FUNCTION_BLOCK "FB_Betr_Std_Zaehl"
TITLE =Betriebsstundenzähler
//KNOW_HOW_PROTECT
//KNOW_HOW_PROTECT
//
//Autor: Ronald Kleißler
//Stand: August 2005
//
//*******************************************************************************
//Eingänge:
//
//Reset:               Setzt den "Btr_Std_Zaehl" auf Null
//Start_Stop:          Startet bzw. stopt den "Btr_Std_Zaehl"
//Takt_MB_aus_der_CPU: Hier wird das MB aus der HW Konfig. der CPU eintragen
//
//Ausgang:
//
//Betr_STD_Zaehler:    Es wird ein DWORD Speicherbereich benötigt
//*******************************************************************************
AUTHOR : 'Kleißler'
NAME : Bter_Std
VERSION : 0.1


VAR_INPUT
  Reset : BOOL ;
  Start_Stop : BOOL ;
  Takt_MB_aus_der_CPU : BYTE ;
END_VAR
VAR_OUTPUT
  Betr_STD_Zaehler : DWORD ;
END_VAR
VAR
  Flankenmerker : BYTE ;
  Minutenimpuls : BOOL ;
  Stundenimpuls : BOOL ;
  Sekunden : INT ;
  Minuten : INT ;
END_VAR
VAR_TEMP
  TEMP0 : BYTE ;
END_VAR
BEGIN
NETWORK
TITLE =Betriebsstundenzähler rücksetzen

      U     #Start_Stop; //*** Betr. Std. Zaehler reseten ***
      SPBN  M100;
      L     0;
      T     #Betr_STD_Zaehler;
      T     #Minuten;
      T     #Sekunden;
      BEB   ;
M100: NOP   0;
NETWORK
TITLE =Betriebsstundenzähler starten bzw. stoppen

      U     #Reset; //*** Betr. Std. Zaehler starten ***
      SPBN  M601;
NETWORK
TITLE =Impuls bilden aus HW Takt
//Erkennung der positiven Flanken des HW Taktes durch die
//XOW (EXKLUSIV-ODER-Wort 16Bit)
//und die UW (UND-Wort 16 Bit) Verknüpfung
      L     #Takt_MB_aus_der_CPU; //Flankenbildung des HW Taktes
      L     #Flankenmerker;
      XOW   ; //XOW Erkennt den Signalwechsel
      UW    ; //UW bildet die Flanke des MB
      T     #TEMP0;
      TAK   ; //Ergebniss aus AKKU 2 nach AKKU 1
      T     #Flankenmerker;
NETWORK
TITLE =Minuten -  Takt
//Addition des Sekundentakt bis 60
      UN    L      0.4; //Flankenpuls einer Sekunden
      SPB   M400; //wenn nein dann Sprung
      L     #Sekunden; //wenn ja dann addition
      +     1;
      T     #Sekunden;
M400: L     #Sekunden; //60 Sekunden erreicht ?
      L     60;
      >=I   ;
      =     #Minutenimpuls; //wenn ja dann plus 1 Minute
      SPBN  M401; //wenn nein dann Spung
      L     0; //wenn ja dann loesche Sekundenzaehler
      T     #Sekunden;
M401: NOP   0;
NETWORK
TITLE =Stunden -  Takt
//Addition des Minutentakt bis 60
      UN    #Minutenimpuls; //Flankenpuls einer Minute
      SPB   M500; //wenn nein dann Sprung
      L     #Minuten; //wenn ja dann addition
      +     1;
      T     #Minuten;
M500: L     #Minuten; //60 Minuten erreicht ?
      L     60;
      >=I   ;
      =     #Stundenimpuls; //wenn ja dann plus 1 Stunde
      SPBN  M501; //wenn nein dann Spung
      L     0; //wenn ja dann loesche Minutenzaehler
      T     #Minuten;
M501: NOP   0;
NETWORK
TITLE =Betriebsstundenzähler
//Freigabe des Betr.-Std.-Zählers über die Verknüpfung in NW 2
      UN    #Stundenimpuls; //Flankenpuls einer Stunde
      SPB   M600; //wenn nein dann Sprung
      L     #Betr_STD_Zaehler; //wenn ja dann addition
      +     1;
      T     #Betr_STD_Zaehler; //Betr. Std. Zaehler Wert
M600: NOP   0;
M601: NOP   0;
END_FUNCTION_BLOCK

